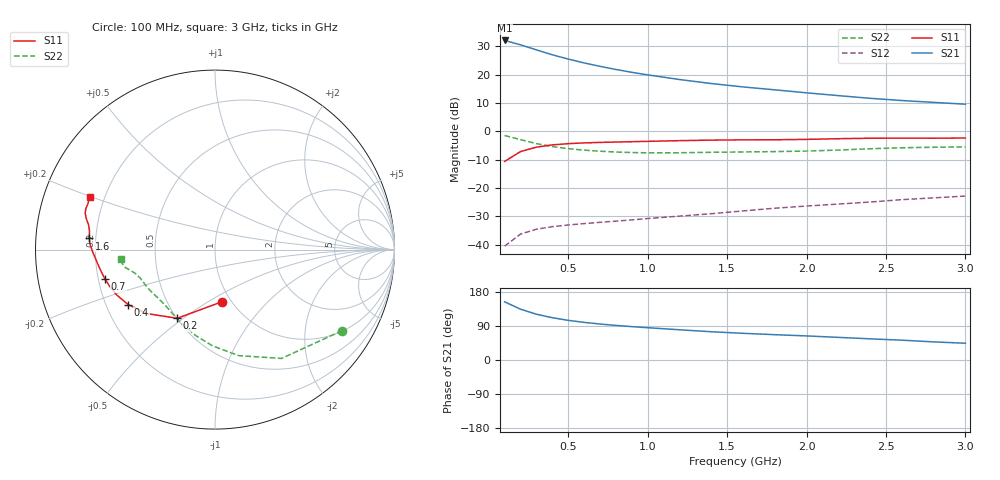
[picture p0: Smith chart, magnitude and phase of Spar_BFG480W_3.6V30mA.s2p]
! Filename: 3_630BFG480.001
! Title: BFG480W
! Bias: Vce=3.6V; Ic=30mA
! Company: NXP Semiconductors NL
! User: Quality&Reliability T&D
! Measure time: 10 Nov 1999 / 11:59:35
#  MHz  S  MA  R 50
! Freq  S11  S21  S12  S22  :
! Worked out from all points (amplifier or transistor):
!   20 points, 100 MHz to 3 GHz, reference 50 ohm
!   highest |S21| = 32.0 dB at 100 MHz (marker M1)
!   |S21| within 3 dB of that: start of sweep to 282.1 MHz
!   unconditionally stable (mu >= 1): 1.169 GHz to end of sweep
!   at 400 MHz: K = 0.50, MSG = 30.3 dB, |S12| = -33.7 dB
!   at 1.2 GHz: K = 1.01, MAG = 23.5 dB, |S12| = -30.0 dB
!   at 3 GHz: K = 1.08, MAG = 14.5 dB, |S12| = -22.9 dB
!   S11 on the Smith chart (normalised r, x): 100 MHz: 0.91, -0.58; 200 MHz: 0.50, -0.47; 400 MHz: 0.29, -0.27; 700 MHz: 0.23, -0.13; 1.6 GHz: 0.17, +0.04; 3 GHz: 0.14, +0.20
100  0.2928 -82.0  39.93 153.6  0.00936 65.5  0.84 -32.5
200  0.4366 -118.8  33.46 134.1  0.01531 54.7  0.7107 -58.6
300  0.5236 -137.2  27.25 120.8  0.01863 48.6  0.6051 -77.5
400  0.5727 -147.7  22.32 111.6  0.02067 46.3  0.5366 -91.4
500  0.6031 -155.2  18.77 104.7  0.02214 45.5  0.4925 -102.2
600  0.6215 -160.7  16.04 99.3  0.0234 46.2  0.4634 -110.5
700  0.6339 -164.9  13.95 95.0  0.02464 47.6  0.4433 -117.2
800  0.6439 -168.4  12.3 91.3  0.0259 49.4  0.4294 -122.9
900  0.6531 -171.5  10.95 88.1  0.02721 51.6  0.4205 -127.8
1000  0.6626 -174.3  9.865 85.2  0.02877 53.4  0.4158 -132.3
1200  0.6811 -178.8  8.171 79.8  0.0317 57.0  0.4168 -139.8
1400  0.6956 177.9  6.938 74.6  0.03497 60.1  0.4242 -145.6
1600  0.7038 174.9  6.048 70.4  0.03915 63.0  0.4304 -149.9
1800  0.7063 171.8  5.375 66.8  0.04376 65.5  0.4367 -154.2
2000  0.7171 169.1  4.756 63.5  0.0478 67.5  0.4458 -159.2
2200  0.7375 166.4  4.246 59.7  0.05179 68.7  0.4649 -163.6
2400  0.7512 164.3  3.807 55.8  0.05626 69.3  0.4899 -166.7
2600  0.755 162.4  3.477 52.3  0.06195 69.8  0.5104 -168.8
2800  0.7526 160.0  3.227 47.8  0.06661 69.1  0.5208 -171.0
3000  0.7581 157.2  2.995 44.3  0.07179 69.1  0.5289 -174.2
